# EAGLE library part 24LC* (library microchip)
Serial EEPROM 128 byte/1 K, 2.5 V, dual mode I2C
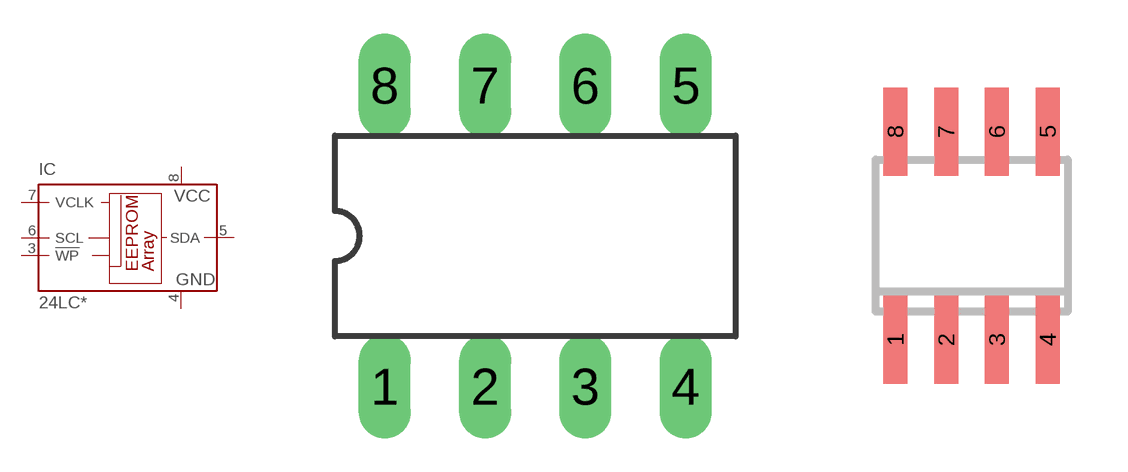
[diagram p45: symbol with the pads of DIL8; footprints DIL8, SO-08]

Designator prefix IC

## 24LCS21AP (MF: MICROCHIP; MPN: 24LCS21A/P; OC_FARNELL: unknown; OC_NEWARK: 92C7023)  [DIL8]
3  !WP  in
4  GND  pwr
5  SDA
6  SCL  in
7  VCLK  in
8  VCC  pwr

## 24LCS21ASN (MF: MICROCHIP; MPN: 24LCS21A/SN; OC_FARNELL: 1847803; OC_NEWARK: 92C7025)  [SO-08]
Pads as for DIL8

## Footprint DIL8 (pad centres in mm)
Dual In Line package type P
drill 0.813 long: 1 -3.81,-3.81; 2 -1.27,-3.81; 3 1.27,-3.81; 4 3.81,-3.81; 5 3.81,3.81; 6 1.27,3.81; 7 -1.27,3.81; 8 -3.81,3.81

## Footprint SO-08 (pad centres in mm)
Small Outline Narrow Plastic Gull Wing 150-mil body, package type SN
smd 0.6 x 2.2: 1 -1.905,-2.6; 2 -0.635,-2.6; 3 0.635,-2.6; 4 1.905,-2.6; 5 1.905,2.6; 6 0.635,2.6; 7 -0.635,2.6; 8 -1.905,2.6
